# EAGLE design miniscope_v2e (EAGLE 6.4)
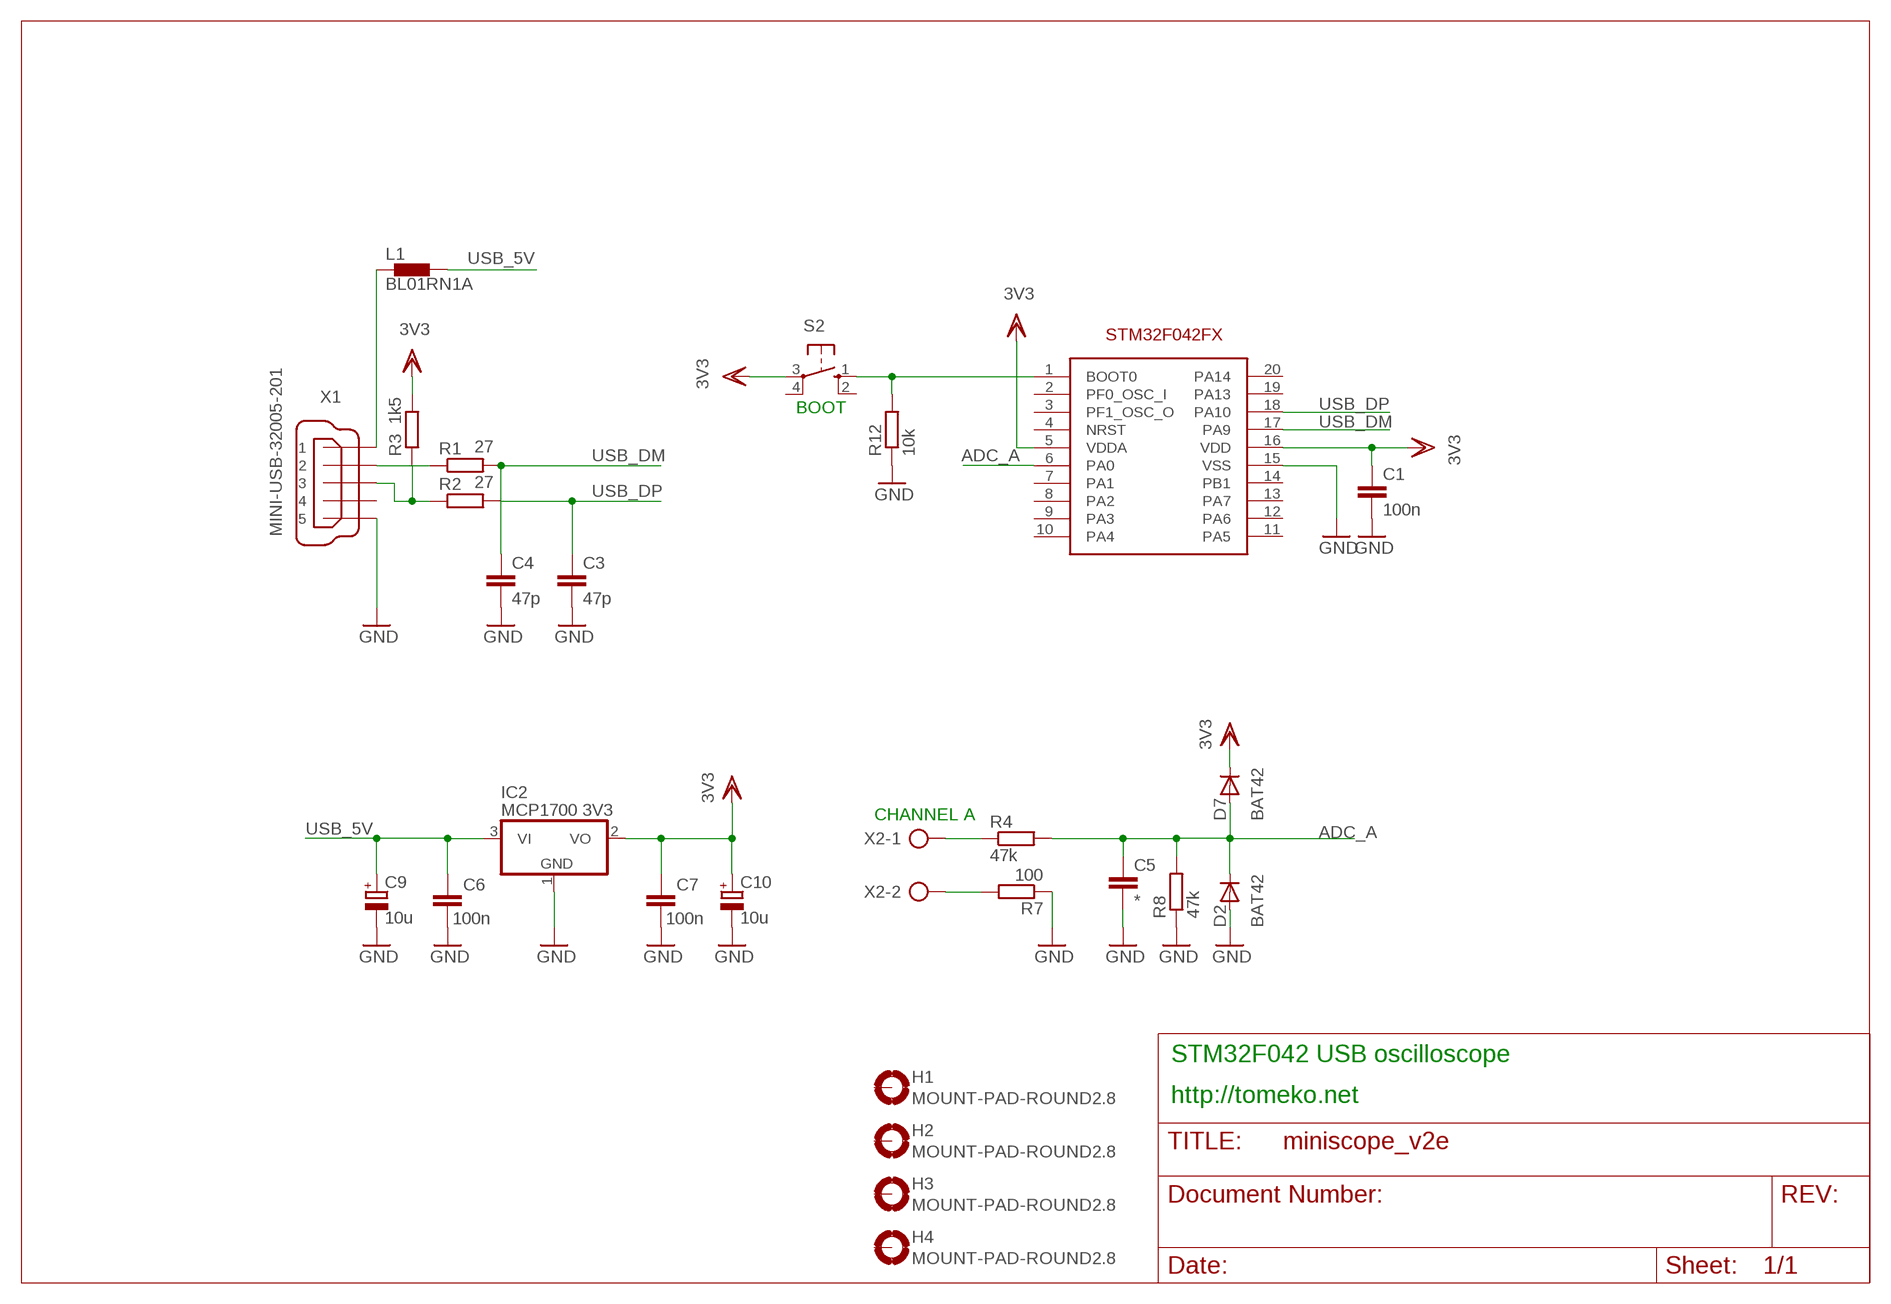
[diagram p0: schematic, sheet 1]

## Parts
C1  100n  C-EUC0805K  [C0805K]
C3  47p  C-EUC0805K  [C0805K]
C4  47p  C-EUC0805K  [C0805K]
C5  *  C-EUC0805K  [C0805K]
C6  100n  C-EUC0805K  [C0805K]
C7  100n  C-EUC0805K  [C0805K]
C9  10u  CPOL-EUCT3216  [CT3216]
C10  10u  CPOL-EUCT3216  [CT3216]
D2  BAT42  1N4148DO35-7  [DO35-7]
D7  BAT42  1N4148DO35-7  [DO35-7]
H1  MOUNT-PAD-ROUND2.8  [2,8-PAD]
H2  MOUNT-PAD-ROUND2.8  [2,8-PAD]
H3  MOUNT-PAD-ROUND2.8  [2,8-PAD]
H4  MOUNT-PAD-ROUND2.8  [2,8-PAD]
IC2  MCP1700 3V3  MCP1703CB  [SOT23]
L1  BL01RN1A  [BL01RN1A]
R1  27  R-EU_R0805  [R0805_40M_SPACE]
R2  27  R-EU_R0805  [R0805_40M_SPACE]
R3  1k5  R-EU_R0805  [R0805_40M_SPACE]
R4  47k  R-EU_R0805  [R0805]
R7  100  R-EU_R0805  [R0805]
R8  47k  R-EU_R0805  [R0805]
R12  10k  R-EU_R0805  [R0805]
S2  10-XX  [B3F-10XX]
U1  STM32F042FX  [TSSOP20]
X1  MINI-USB-32005-201  [32005-201]
X2  AK500/2  [AK500/2]

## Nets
ADC_A: C5.1 D2.C D7.A R4.2 R8.2 U1.6(PA0)
GND: C1.2 C3.2 C4.2 C5.2 C6.1 C7.1 C9.- C10.- D2.A IC2.1(GND) R7.1 R8.1 R12.1 U1.15(VSS) X1.5
N$2: R1.1 X1.2
N$4: L1.1 X1.1
N$5: R2.1 R3.1 X1.3
N$9: R12.2 S2.1(S) U1.1(BOOT0)
N$11: R7.2 X2.2
N$13: R4.1 X2.1
USB_5V: C6.2 C9.+ IC2.3(VI) L1.2
USB_DM: C4.1 R1.2 U1.17(PA9)
USB_DP: C3.1 R2.2 U1.18(PA10)
VDD: C1.1 C7.2 C10.+ D7.C IC2.2(VO) R3.2 S2.3(P) U1.5(VDDA) U1.16(VDD) ; supply symbol labelled 3V3
Unconnected: H1.B2,8(MOUNT) H2.B2,8(MOUNT) H3.B2,8(MOUNT) H4.B2,8(MOUNT) S2.2(S1) S2.4(P1) U1.2(PF0_OSC_I) U1.3(PF1_OSC_O) U1.4(NRST) U1.7(PA1) U1.8(PA2) U1.9(PA3) U1.10(PA4) U1.11(PA5) U1.12(PA6) U1.13(PA7) U1.14(PB1) U1.19(PA13) U1.20(PA14) X1.4

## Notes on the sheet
- BOOT
- CHANNEL A
- STM32F042 USB oscilloscope
- http://tomeko.net

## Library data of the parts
C1 C3-C7 = resistor:C-EU: CAPACITOR, European symbol
C9 C10 = resistor:CPOL-EU: POLARIZED CAPACITOR, European symbol
D2 D7 = diode:1N4148: DIODE
H1-H4 = holes:MOUNT-PAD-ROUND: MOUNTING PAD, round
IC2 = linear:MCP1703: 250 mA, 16V, Low Quiescent Current LDO Regulator Source: http://ww1.microchip.com/downloads/en/DeviceDoc/22049b.pdf
L1 = inductors:BL0: Noise Suppression Products/EMI Suppression Filters, Lead EMIFIL(R) Inductor Type
R1-R3 = resistor:R-EU_: RESISTOR, European symbol
R4 R7 R8 R12 = rcl:R-EU_: RESISTOR, European symbol
S2 = switch-omron:10-XX: OMRON SWITCH; MPN: B3F-1000; OC_FARNELL: 176432; OC_NEWARK: 36M3542
U1 = STM32F042Fx:STM32F042FX: STM32F042Fx microcontroller
X1 = con-cypressindustries:MINI-USB-: MINI USB-B Conector Source: www.cypressindustries.com; OC_FARNELL: unknown; OC_NEWARK: unknown
X2 = con-ptr500:AK500/2: CONNECTOR; OC_FARNELL: unknown; OC_NEWARK: unknown

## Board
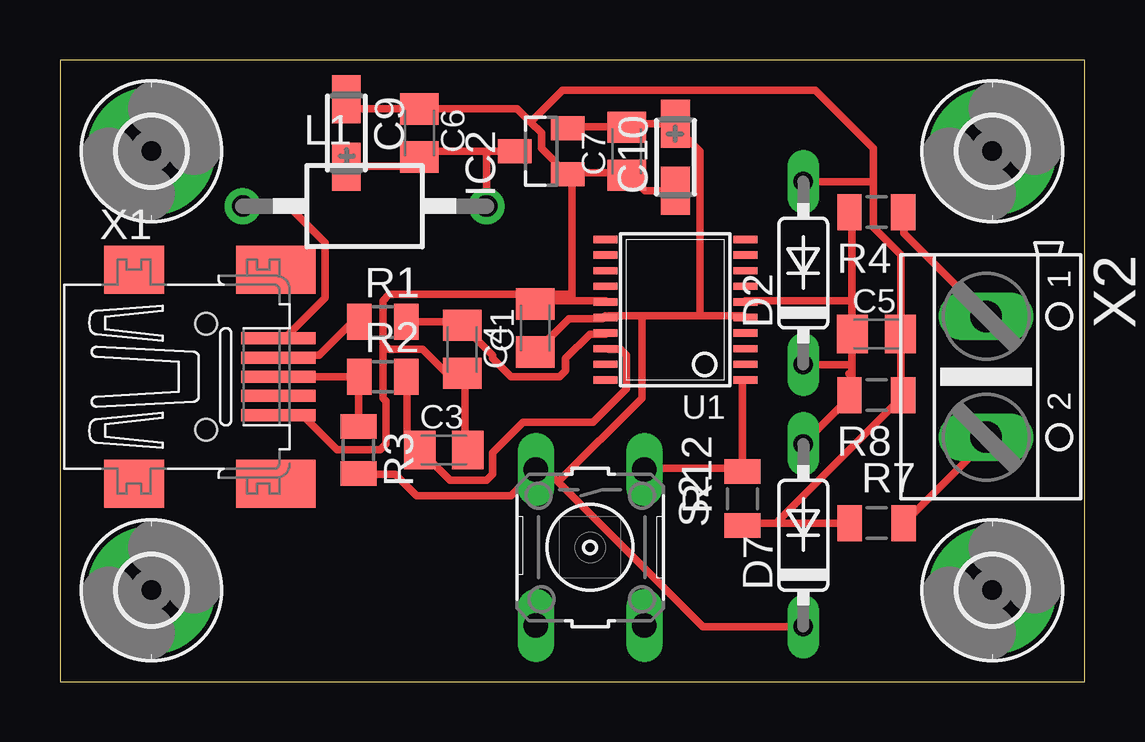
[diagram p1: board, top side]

Size 42.72 x 25.9 mm. Coordinates in mm from the lower left corner, seen from the top.
Outline: 0,0 42.72,0 42.72,25.9 0,25.9 0,0
Copper layers (1*16): Top 0.035mm / dielectric 1.5mm / Bottom 0.035mm
Design rules "default *": minimum track width 12mil, minimum drill 24mil, track to track 10mil, track to pad 9mil, pad to pad 10mil, via to via 10mil, smd to smd 10mil, copper to edge 40mil, drill to drill 8mil, minimum pad ring 10mil, minimum via ring 8mil, stop-mask expansion 4mil, vias tented up to drill 0mil, thermal gap 10mil

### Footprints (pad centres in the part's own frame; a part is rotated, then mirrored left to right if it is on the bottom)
C0805K = smd 1.3 x 1.6: 1 -1,0; 2 1,0
CT3216 = smd 2 x 1.2: + 1.4,0; - -1.4,0
DO35-7 = drill 0.813 long: A 3.81,0; C -3.81,0
2,8-PAD = drill 2.8 pad 5.334: B2,8 0,0
SOT23 = smd 1 x 1.4: 1 -0.95,-1.1; 2 0.95,-1.1; 3 0,1.1
BL01RN1A = drill 0.9 pad 1.5: 1 -5.08,0; 2 5.08,0
R0805_40M_SPACE = smd 1.016 x 1.5: 1 -0.977,0; 2 0.977,0
R0805 = smd 1.016 x 1.5: 1 -1.118,0; 2 1.128,0
B3F-10XX = drill 1.016 long: 1 -3.251,2.261; 2 3.251,2.261; 3 -3.251,-2.261; 4 3.251,-2.261
TSSOP20 = smd 0.305 x 0.991: 1 -2.925,-2.918; 2 -2.275,-2.918; 3 -1.625,-2.918; 4 -0.975,-2.918; 5 -0.325,-2.918; 6 0.325,-2.918; 7 0.975,-2.918; 8 1.625,-2.918; 9 2.275,-2.918; 10 2.925,-2.918; 11 2.925,2.918; 12 2.275,2.918; 13 1.625,2.918; 14 0.975,2.918; 15 0.325,2.918; 16 -0.325,2.918; 17 -0.975,2.918; 18 -1.625,2.918; 19 -2.275,2.918; 20 -2.925,2.918
32005-201 = smd 3.1 x 0.5: 1 3,1.6; 2 3,0.8; 3 3,0; 4 3,-0.8; 5 3,-1.6 | smd 2.5 x 2: M1 -3,-4.45; M2 -3,4.45 | smd 3.3 x 2: M3 2.9,4.45; M4 2.9,-4.45 | hole 0.9: 0,2.2; 0,-2.2
AK500/2 = drill 1.321 long: 1 -2.515,0; 2 2.515,0

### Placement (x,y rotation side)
C1  19.81,14.73 90 top
C3  16,9.65 0 top
C4  16.76,13.84 270 top
C5  34.04,14.48 0 top
C6  14.99,22.86 270 top
C7  23.62,22.1 90 top
C9  11.94,22.86 270 top
C10  25.65,21.84 90 top
D2  30.99,17.02 90 top
D7  30.99,6.1 90 top
H1  3.81,3.81 0 top
H2  3.81,22.1 0 top
H3  38.86,22.1 0 top
H4  38.86,3.81 0 top
IC2  20.07,22.1 90 top
L1  12.7,19.81 0 top
R1  13.46,14.99 0 top
R2  13.46,12.7 0 top
R3  12.45,9.65 270 top
R4  34.04,19.56 180 top
R7  34.04,6.6 0 top
R8  34.04,11.94 180 top
R12  28.45,7.62 90 top
S2  22.1,5.59 270 top
U1  25.65,15.49 90 top
X1  6.1,12.7 0 top
X2  38.61,12.7 270 top

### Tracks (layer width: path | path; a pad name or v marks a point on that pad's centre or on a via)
ADC_A
  Top 0.305: 33.02,13.21 33.02,14.48 C5.1 33.02,14.61 33.02,15.88 | 33.02,13.21 33.02,12.83 | 33.02,12.83 33.02,11.94 R8.2 32.89,11.81 D7.A | 33.02,15.88 33.02,19.56 R4.2 | 32.89,12.83 33.02,12.83 | 33.02,15.88 28.57,15.88 U1.6 | D2.C 33.02,13.21
GND
  Top 0.305: C9.- 12.32,23.88 14.99,23.88 C6.1 15.11,23.88 19.05,23.88 19.62,23.3 | C3.2 16.89,9.65 16.89,12.7 16.76,12.83 C4.2 16.64,12.83 16.13,12.83 15.11,13.84 13.72,13.84 13.53,14.03 | 21.34,15.88 19.94,15.88 19.81,15.75 C1.2 | 21.34,15.88 22.73,15.88 U1.15 | IC2.1 21.21,21.21 23.62,21.21 C7.1 23.75,21.08 24.38,20.45 C10.- | 21.34,16.13 21.34,21.08 IC2.1 | 21.34,16.13 21.34,15.88 | 13.53,14.03 13.46,14.1 13.46,15.88 13.72,16.13 21.34,16.13 | 19.62,23.3 20.07,22.86 20.07,22.23 21.08,21.21 IC2.1 | X1.5 9.14,11.05 10.16,11.05 11.56,9.65 13.34,9.65 13.59,9.91 13.59,11.68 13.46,11.81 13.46,13.97 13.53,14.03 | 33.91,20.83 33.91,22.23 31.5,24.64 20.95,24.64 19.62,23.3 | 33.91,20.83 33.91,18.92 35.05,17.78 35.05,14.61 C5.2 35.05,14.48 35.05,11.94 R8.1 35.05,11.81 29.97,6.73 29.97,6.6 | 33.91,20.83 D2.A | R7.1 29.97,6.6 | 29.97,6.6 28.45,6.6 R12.1
N$2
  Top 0.305: R1.1 12.19,14.99 10.79,13.59 9.14,13.59 X1.2
N$4
  Top 0.305: L1.1 9.53,19.81 11.05,18.29 11.05,16 9.4,14.35 9.14,14.35 X1.1
N$5
  Top 0.305: R3.1 12.45,12.7 R2.1 X1.3
N$9
  Top 0.305: U1.1 28.45,12.45 R12.2 28.32,8.89 24.38,8.89 S2.1
N$11
  Top 0.305: X2.2 38.61,10.03 35.18,6.6 R7.2
N$13
  Top 0.305: R4.1 35.18,19.56 35.18,18.67 38.61,15.24 X2.1
USB_5V
  Top 0.305: 14.99,21.97 C6.2 | C9.+ 14.48,21.46 14.86,21.84 C6.2 | 17.78,22.1 14.99,22.1 C6.2 | 17.78,22.1 IC2.3 | L1.2 17.78,22.1
USB_DM
  Top 0.305: U1.17 22.73,14.48 22.1,14.48 21.08,13.46 21.08,12.95 20.83,12.7 18.8,12.7 18.03,13.46 18.03,13.59 16.76,14.86 C4.1 16.76,14.99 R1.2
USB_DP
  Top 0.305: U1.18 22.86,13.84 23.37,13.84 23.62,13.59 23.62,12.19 22.23,10.79 19.3,10.79 18.03,9.53 18.03,8.64 17.78,8.38 16.26,8.38 14.99,9.65 C3.1 14.99,9.78 14.48,10.29 14.48,12.7 R2.2
VDD
  Top 0.305: 22.73,15.24 U1.16 | U1.16 22.61,15.11 21.21,15.11 19.81,13.72 C1.1 | R3.2 12.45,8.64 13.97,8.64 14.86,7.75 18.8,7.75 19.81,8.76 S2.3 19.94,8.76 20.32,8.76 20.77,8.32 | IC2.2 21.21,23.11 23.62,23.11 C7.2 23.62,23.24 C10.+ 25.65,23.11 26.67,22.1 26.67,15.24 | 24.26,15.24 22.86,15.24 U1.16 | 24.26,15.24 26.67,15.24 | 26.67,15.24 28.45,15.24 U1.5 | D7.C 26.8,2.29 20.77,8.32 | 24.26,15.24 24.26,11.81 20.77,8.32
